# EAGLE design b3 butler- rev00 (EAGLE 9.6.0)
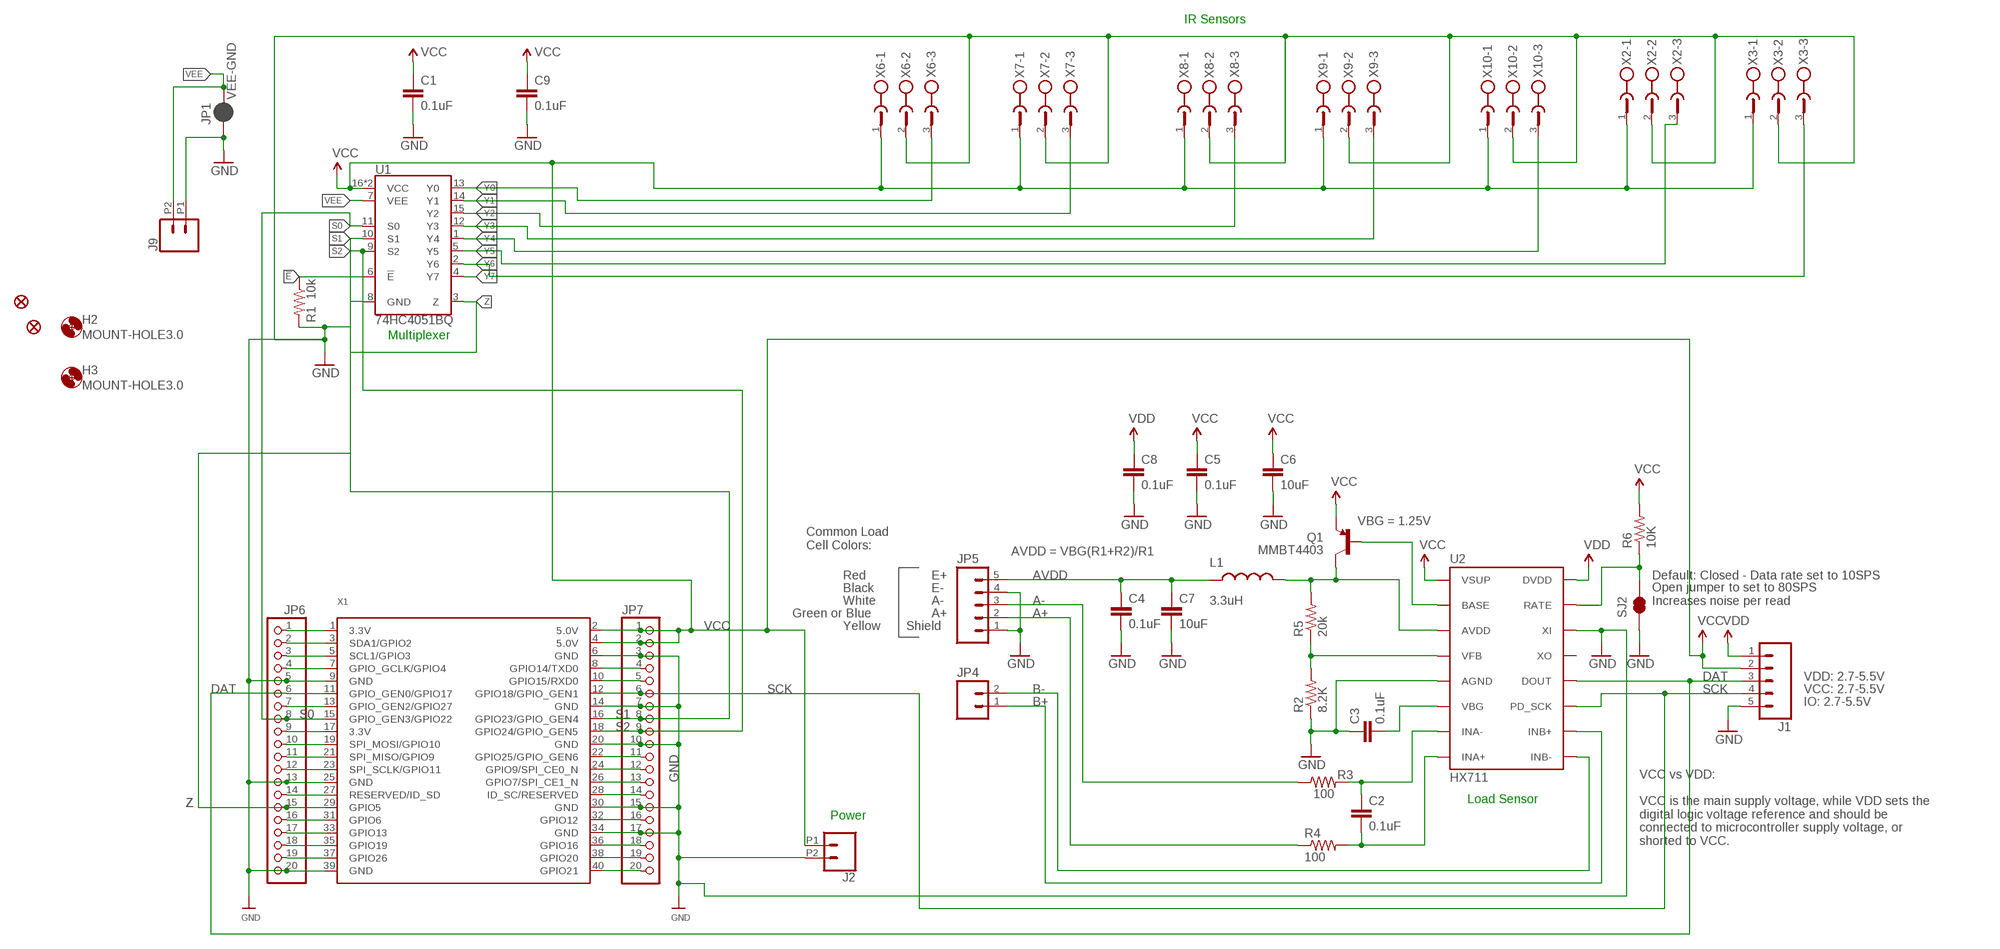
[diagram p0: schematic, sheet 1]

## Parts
C1  0.1uF  0.1UF-0603-25V-(+80/-20%)  [0603]
C2  0.1uF  0.1UF-25V-5%(0603)  [0603-CAP]
C3  0.1uF  0.1UF-25V-5%(0603)  [0603-CAP]
C4  0.1uF  0.1UF-25V-5%(0603)  [0603-CAP]
C5  0.1uF  0.1UF-25V-5%(0603)  [0603-CAP]
C6  10uF  10UF50V20%(1210)  [1210]
C7  10uF  10UF50V20%(1210)  [1210]
C8  0.1uF  0.1UF-25V-5%(0603)  [0603-CAP]
C9  0.1uF  0.1UF-0603-25V-(+80/-20%)  [0603]
FD1  FIDUCIAL1X2  [FIDUCIAL-1X2]
FD2  FIDUCIAL1X2  [FIDUCIAL-1X2]
H2  MOUNT-HOLE3.0  [3,0]
H3  MOUNT-HOLE3.0  [3,0]
J1  M05PTH  [1X05]
J2  CONN_022.54MM_SCREWTERM  [1X02_2.54_SCREWTERM]
J9  CONN_022.54MM_SCREWTERM  [1X02_2.54_SCREWTERM]
JP1  VEE-GND  JUMPER-PAD-2-NC_BY_PASTENO-SILK  [PAD-JUMPER-2-NC_BY_PASTE_NO_SILK]
JP4  M02PTH  [1X02@1]
JP5  M05PTH  [1X05]
JP6  HEADER-1X20ROUND  [1X20_ROUND]
JP7  HEADER-1X20ROUND  [1X20_ROUND]
L1  3.3uH  INDUCTOR0805-IND  [0805]
Q1  MMBT4403  TRANSISTOR_PNPMMBT4403  [SOT23-3]
R1  10k  10KOHM-0603-1/10W-1%  [0603]
R2  8.2K  8.2KOHM-1/10W-5%(0603)  [0603-RES]
R3  100  100OHM-1/10W-1%(0603)  [0603-RES]
R4  100  100OHM-1/10W-1%(0603)  [0603-RES]
R5  20k  20KOHM1/10W1%(0603)  [0603-RES]
R6  10K  10KOHM-1/10W-1%(0603)0603  [0603-RES]
SJ2  JUMPER-PAD-2-NC_BY_TRACE  [PAD-JUMPER-2-NC_BY_TRACE_YES_SILK]
U1  74HC4051BQ  [DHVQFN-16-2.5X3.5MM]
U2  HX711  HX711HX711  [SO16]
X1  RASPBERRYPI_B+_IDC  [RASPBERRYPI_B+_IDC]
X2  W232-3  [W232-3]
X3  W232-3  [W232-3]
X6  W232-3  [W232-3]
X7  W232-3  [W232-3]
X8  W232-3  [W232-3]
X9  W232-3  [W232-3]
X10  W232-3  [W232-3]

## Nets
!E!: R1.1 U1.6(!E!)
A+: JP5.2 R4.1
A-: JP5.3 R3.1
AVDD [POWER]: C4.1 C7.1 JP5.5 L1.1
B+: JP4.1 U2.10(INB+)
B-: JP4.2 U2.9(INB-)
DAT: J1.3 JP6.6 U2.12(DOUT) X1.11(GPIO_GEN0/GPIO17)
GND [POWER]: C1.2 C3.1 C4.2 C5.2 C6.2 C7.2 C8.2 C9.2 J1.5 J2.P2 J9.P1 JP1.1 JP5.1 JP5.4 JP6.5 JP6.13 JP6.20 JP7.3 JP7.7 JP7.10 JP7.15 JP7.17 R1.2 R2.1 SJ2.1 U1.8(GND) U2.5(AGND) U2.14(XI) X1.6(GND) X1.9(GND) X1.14(GND) X1.20(GND) X1.25(GND) X1.30(GND) X1.34(GND) X1.39(GND) X2.2 X3.2 X6.2 X7.2 X8.2 X9.2 X10.2
N$1: R6.1 SJ2.2 U2.15(RATE)
N$2: C2.1 R3.2 U2.7(INA-)
N$3: C2.2 R4.2 U2.8(INA+)
N$4: Q1.1(B) U2.2(BASE)
N$5: L1.2 Q1.3(C) R5.2 U2.3(AVDD)
N$6: R2.2 R5.1 U2.4(VFB)
N$7: C3.2 U2.6(VBG)
N$11: JP7.4 X1.8(GPIO14/TXD0)
N$12: JP7.5 X1.10(GPIO15/RXD0)
N$16: JP7.11 X1.22(GPIO25/GPIO_GEN6)
N$17: JP7.12 X1.24(GPIO9/SPI_CE0_N)
N$18: JP7.13 X1.26(GPIO7/SPI_CE1_N)
N$19: JP7.14 X1.28(ID_SC/RESERVED)
N$20: JP7.16 X1.32(GPIO12)
N$21: JP7.18 X1.36(GPIO16)
N$22: JP7.19 X1.38(GPIO20)
N$23: JP7.20 X1.40(GPIO21)
N$24: JP6.1 X1.1(3.3V)
N$25: JP6.2 X1.3(SDA1/GPIO2)
N$26: JP6.3 X1.5(SCL1/GPIO3)
N$27: JP6.4 X1.7(GPIO_GCLK/GPIO4)
N$29: JP6.7 X1.13(GPIO_GEN2/GPIO27)
N$31: JP6.9 X1.17(3.3V)
N$32: JP6.10 X1.19(SPI_MOSI/GPIO10)
N$33: JP6.11 X1.21(SPI_MISO/GPIO9)
N$34: JP6.12 X1.23(SPI_SCLK/GPIO11)
N$35: JP6.14 X1.27(RESERVED/ID_SD)
N$37: JP6.16 X1.31(GPIO6)
N$38: JP6.17 X1.33(GPIO13)
N$39: JP6.18 X1.35(GPIO19)
N$40: JP6.19 X1.37(GPIO26)
S0: JP6.8 U1.11(S0) X1.15(GPIO_GEN3/GPIO22)
S1: JP7.8 U1.10(S1) X1.16(GPIO23/GPIO_GEN4)
S2: JP7.9 U1.9(S2) X1.18(GPIO24/GPIO_GEN5)
SCK: J1.4 JP7.6 U2.11(PD_SCK) X1.12(GPIO18/GPIO_GEN1)
VCC [IR SENSORS]: C1.1 C5.1 C6.1 C9.1 J1.2 J2.P1 JP7.1 JP7.2 Q1.2(E) R6.2 U1.16(VCC) U1.EP(VCC) U2.1(VSUP) X1.2(5.0V) X1.4(5.0V) X2.1 X3.1 X6.1 X7.1 X8.1 X9.1 X10.1
VDD [POWER]: C8.1 J1.1 U2.16(DVDD)
VEE [POWER]: J9.P2 JP1.2 U1.7(VEE)
Y0 [IR SENSORS]: U1.13(Y0) X6.3
Y1 [IR SENSORS]: U1.14(Y1) X7.3
Y2 [IR SENSORS]: U1.15(Y2) X8.3
Y3 [IR SENSORS]: U1.12(Y3) X9.3
Y4 [IR SENSORS]: U1.1(Y4) X10.3
Y5 [IR SENSORS]: U1.5(Y5) X2.3
Y6 [IR SENSORS]: U1.2(Y6) X3.3
Y7 [IR SENSORS]: U1.4(Y7)
Z: JP6.15 U1.3(Z) X1.29(GPIO5)
Unconnected: U2.13(XO)

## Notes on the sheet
- IR Sensors
- Multiplexer
- VBG = 1.25V
- Common Load
  Cell Colors:
- AVDD = VBG(R1+R2)/R1
- Red | E+ | Default: Closed - Data rate set to 10SPS
- Black | E-
- White | A-
- Open jumper to set to 80SPS
  Increases noise per read
- Green or Blue | A+
- Yellow | Shield
- VDD: 2.7-5.5V
- VCC: 2.7-5.5V
- IO: 2.7-5.5V
- Load Sensor
- Power
- VCC vs VDD:
  
  VCC is the main supply voltage, while VDD sets the
  digital logic voltage reference and should be
  connected to microcontroller supply voltage, or
  shorted to VCC.

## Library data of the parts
C1 C9 = SparkFun-Capacitors:0.1UF: 0.1µF ceramic capacitors; PROD_ID: CAP-00810
C2-C5 C8 = SparkFun-Capacitors:0.1UF-25V-5%(0603): CAP-08604; PROD_ID: CAP-08604
C6 C7 = SparkFun-Capacitors:10UF50V20%(1210): CAP-09824; PROD_ID: CAP-09824
FD1 FD2 = SparkFun-Aesthetics:FIDUCIAL: Fiducial Alignment Points
H2 H3 = holes:MOUNT-HOLE: MOUNTING HOLE with drill center marker
J1 JP5 = SparkFun-Connectors:M05: Header 5 Standard 5-pin 0.1" header. Use with straight break away headers (SKU : PRT-00116), right angle break away headers (PRT-00553), swiss pins (PRT-00743), machine pins (PRT-00117), and female headers (PRT-00115). Molex polarized connector foot print use with SKU : PRT-08230 with associated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
J2 J9 = SparkFun-Connectors:CONN_02: Multi connection point. Often used as Generic Header-pin footprint for 0.1 inch spaced/style header connections
JP1 = SparkFun-Passives:JUMPER-PAD-2-NC_BY_PASTE
JP4 = SparkFun-Connectors:M02: Standard 2-pin 0.1" header. Use with
JP6 JP7 = microbuilder:HEADER-1X20
L1 = SparkFun-Passives:INDUCTOR: Inductors; PROD_ID: NDUC-13076
Q1 = SparkFun-DiscreteSemi:TRANSISTOR_PNP: Generic PNP BJT Double check pinouts against datasheets- not all devices are the same! MMBT3906 - 40V 200mA SOT-23 (TRANS-08052) MMBT4403 - 40V 600mA SOT-23 (TRANS-09245); PROD_ID: TRANS-09245
R1 = SparkFun-Resistors:10KOHM: 10kΩ resistor; PROD_ID: RES-00824
R2 = SparkFun-Resistors:8.2KOHM-1/10W-5%(0603): RES-10646; PROD_ID: RES-10646
R3 R4 = SparkFun-Resistors:100OHM-1/10W-1%(0603): RES-07863; PROD_ID: RES-07863
R5 = SparkFun-Resistors:20KOHM1/10W1%(0603): RES-09383; PROD_ID: RES-09383
R6 = SparkFun-Resistors:10KOHM-1/10W-1%(0603): RES-00824; PROD_ID: RES-00824
SJ2 = SparkFun-Passives:JUMPER-PAD-2-NC_BY_TRACE
U1 = 8mux:74HC4051: NXP 74HC4051 8-Channel Analog Multiplexer/Demultiplexer The 74HC4051; 74HCT4051 is a single-pole octal-throw analog switch (SP8T) suitable for use in analog or digital 8:1 multiplexer/demultiplexer applications. The switch features three digital select inputs (S0, S1 and S2), eight independent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; PROD_ID: IC-13334
U2 = Testing:HX711; PROD_ID: IC-12445
X1 = microbuilder:RASPBERRYPI_B+_IDC
X2 X3 X6-X10 = con-wago-508:W232-3: WAGO SREW CLAMP; OC_FARNELL: unknown; OC_NEWARK: unknown

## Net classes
0 default: width 0.203 mm, drill 0.406 mm, clearance 0.203 mm
1 POWER: width 0.813 mm, drill 0.406 mm, clearance 0.203 mm
2 IR SENSORS: width 0.203 mm, drill 0.203 mm, clearance 0.152 mm

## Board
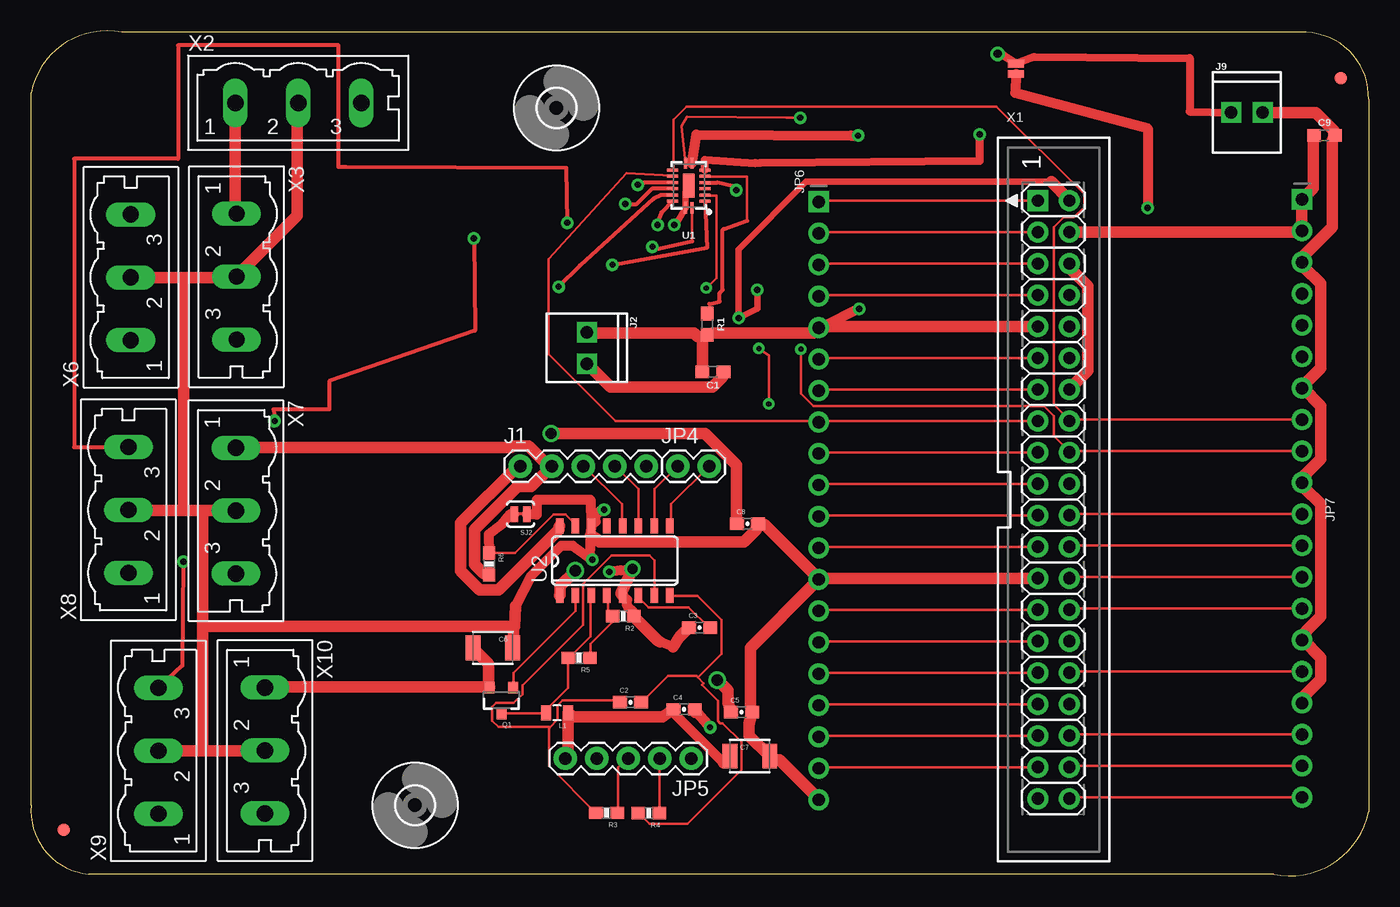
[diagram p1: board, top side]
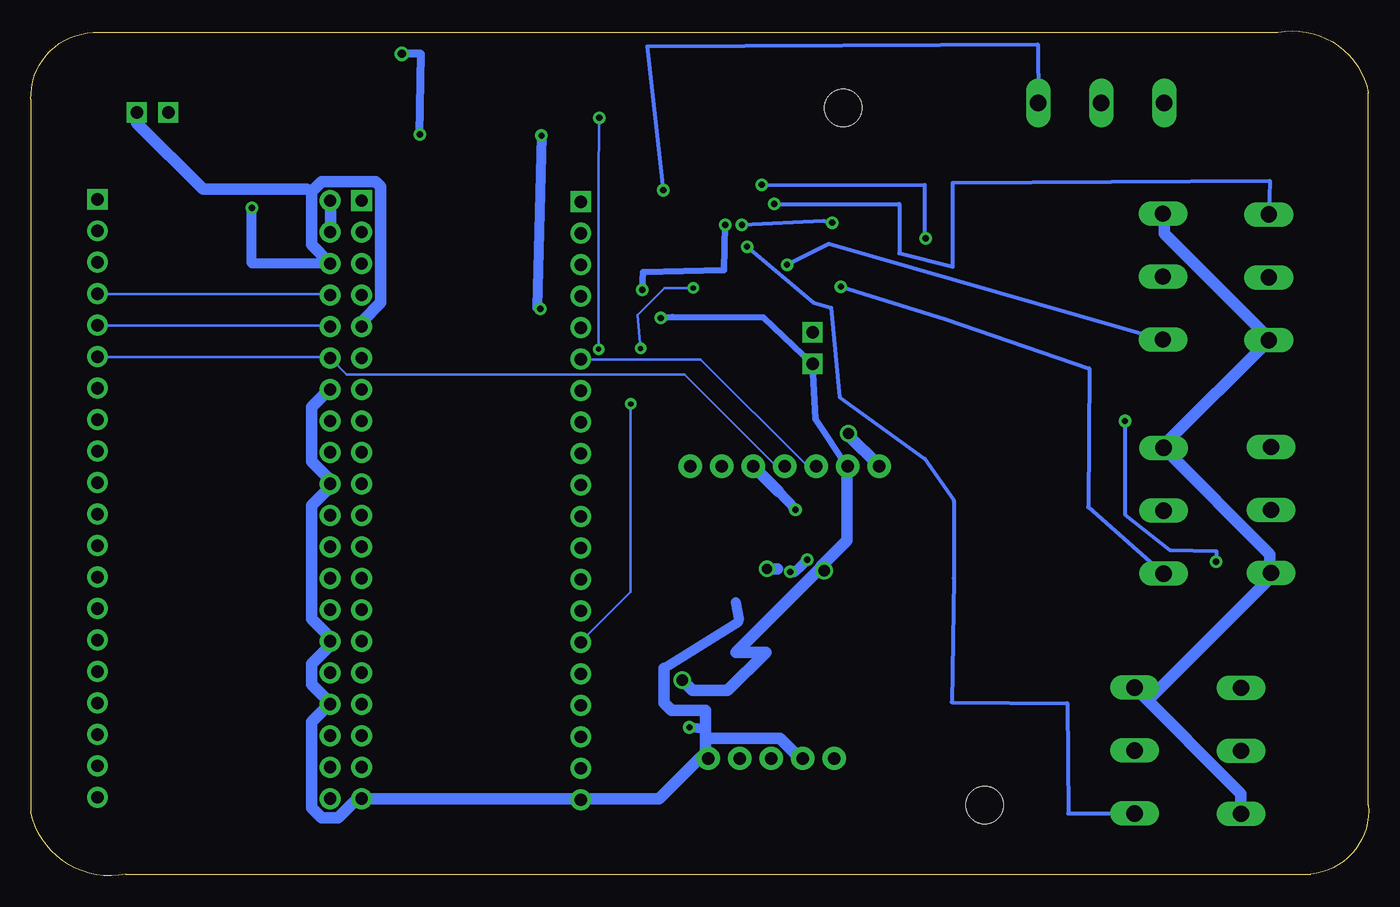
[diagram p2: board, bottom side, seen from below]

Size 107.91 x 68.17 mm. Coordinates in mm from the lower left corner, seen from the top.
Outline: 107.91,62.65 107.91,5.15 arc-90 100.26,0.13 4.66,0.13 arc-90 0.02,5.7 0.02,63.2 arc-90 7.3,68.05 102.9,68.05 arc-90 107.91,62.65
Copper layers (1*16): Top 0.035mm / dielectric 1.5mm / Bottom 0.035mm
Design rules "SparkFun": minimum track width 8mil, minimum drill 20mil, track to track 8mil, track to pad 8mil, pad to pad 8mil, via to via 8mil, smd to smd 8mil, copper to edge 8mil, drill to drill 8mil, minimum pad ring 12mil, minimum via ring 10mil, stop-mask expansion 4mil, vias tented up to drill 20mil, thermal gap 10mil

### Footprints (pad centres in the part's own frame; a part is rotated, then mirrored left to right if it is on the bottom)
0603 = smd 1.1 x 1: 1 -0.85,0; 2 0.85,0
0603-CAP = smd 1.1 x 1: 1 -0.85,0; 2 0.85,0
1210 = smd 1.2 x 2: 1 -1.6,0; 2 1.6,0
FIDUCIAL-1X2 = smd 1 x 1: 1 0,0
3,0 = hole 3: 0,0
1X05 = drill 1.016 pad 1.88: 1 0,0; 2 2.54,0; 3 5.08,0; 4 7.62,0; 5 10.16,0
1X02_2.54_SCREWTERM = drill 1.016 square: P1 2.54,0; P2 0,0
PAD-JUMPER-2-NC_BY_PASTE_NO_SILK = smd 0.635 x 1.27: 1 -0.401,0; 2 0.413,0
1X02@1 = drill 1.016 pad 1.88: 1 0,0; 2 2.54,0
1X20_ROUND = drill 1 pad 1.676 square: 1 -24.13,0 | drill 1 pad 1.676: 2 -21.59,0; 3 -19.05,0; 4 -16.51,0; 5 -13.97,0; 6 -11.43,0; 7 -8.89,0; 8 -6.35,0; 9 -3.81,0; 10 -1.27,0; 11 1.27,0; 12 3.81,0; 13 6.35,0; 14 8.89,0; 15 11.43,0; 16 13.97,0; 17 16.51,0; 18 19.05,0; 19 21.59,0; 20 24.13,0
0805 = smd 0.8 x 1.2: 1 -0.9,0; 2 0.9,0
SOT23-3 = smd 0.8 x 0.9: 1 -0.95,-1; 2 0.95,-1; 3 0,1.1
0603-RES = smd 1.1 x 1: 1 -0.85,0; 2 0.85,0
PAD-JUMPER-2-NC_BY_TRACE_YES_SILK = smd 0.635 x 1.27: 1 -0.508,0; 2 0.508,0
DHVQFN-16-2.5X3.5MM = smd 0.9 x 0.24: 1 -1.8,-0.25; 8 1.8,-0.25; 9 1.8,0.25; 16 -1.8,0.25 | smd 0.24 x 0.9: 2 -1.25,-1.3; 3 -0.75,-1.3; 4 -0.25,-1.3; 5 0.25,-1.3; 6 0.75,-1.3; 7 1.25,-1.3; 10 1.25,1.3; 11 0.75,1.3; 12 0.25,1.3; 13 -0.25,1.3; 14 -0.75,1.3; 15 -1.25,1.3 | smd 1.9 x 0.9: EP 0,0
SO16 = smd 0.6 x 1.2: 1 -4.445,-2.8; 2 -3.175,-2.8; 3 -1.905,-2.8; 4 -0.635,-2.8; 5 0.635,-2.8; 6 1.905,-2.8; 7 3.175,-2.8; 8 4.445,-2.8; 9 4.445,2.8; 10 3.175,2.8; 11 1.905,2.8; 12 0.635,2.8; 13 -0.635,2.8; 14 -1.905,2.8; 15 -3.175,2.8; 16 -4.445,2.8
RASPBERRYPI_B+_IDC = drill 1 pad 1.676 square: 1 -1.27,24.13 | drill 1 pad 1.676: 2 1.27,24.13; 3 -1.27,21.59; 4 1.27,21.59; 5 -1.27,19.05; 6 1.27,19.05; 7 -1.27,16.51; 8 1.27,16.51; 9 -1.27,13.97; 10 1.27,13.97; 11 -1.27,11.43; 12 1.27,11.43; 13 -1.27,8.89; 14 1.27,8.89; 15 -1.27,6.35; 16 1.27,6.35; 17 -1.27,3.81; 18 1.27,3.81; 19 -1.27,1.27; 20 1.27,1.27; 21 -1.27,-1.27; 22 1.27,-1.27; 23 -1.27,-3.81; 24 1.27,-3.81; 25 -1.27,-6.35; 26 1.27,-6.35; 27 -1.27,-8.89; 28 1.27,-8.89; 29 -1.27,-11.43; 30 1.27,-11.43; 31 -1.27,-13.97; 32 1.27,-13.97; 33 -1.27,-16.51; 34 1.27,-16.51; 35 -1.27,-19.05; 36 1.27,-19.05; 37 -1.27,-21.59; 38 1.27,-21.59; 39 -1.27,-24.13; 40 1.27,-24.13
W232-3 = drill 1.321 long: 1 -5.08,-0.635; 2 0,-0.635; 3 5.08,-0.635

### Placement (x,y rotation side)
C1  55.02,40.67 180 top
C2  48.37,14 0 top
C3  53.94,20.03 0 top
C4  52.69,13.43 0 top
C5  57.33,13.2 0 top
C6  37.26,18.38 0 top
C7  58,9.66 0 top
C8  57.81,28.41 0 top
C9  104.35,59.73 0 top
FD1  105.65,64.37 0 top
FD2  2.65,3.72 0 top
H2  42.4,61.96 0 top
H3  30.98,5.69 0 top
J1  39.48,33.05 0 top
J2  44.85,43.85 270 top
J9  96.83,61.59 0 top
JP1  79.46,65.11 90 top
JP4  52.18,33.05 0 top
JP5  53.26,9.47 180 top
JP6  63.55,30.26 270 top
JP7  102.55,30.46 270 top
L1  42.44,13.15 180 top
Q1  37.95,14.19 180 top
R1  54.57,44.51 270 top
R2  47.79,20.94 180 top
R3  46.44,5.08 180 top
R4  49.85,5.06 180 top
R5  44.22,17.59 180 top
R6  36.96,25.17 270 top
SJ2  39.5,29.18 180 top
U1  53.07,55.69 90 top
U2  47.1,25.43 0 top
X1  82.5,30.35 0 top
X2  21.57,63 0 top
X3  17.22,48.35 270 top
X6  7.41,48.29 90 top
X7  17.17,29.46 270 top
X8  7.22,29.52 90 top
X9  9.64,10.08 90 top
X10  19.52,10.11 270 top

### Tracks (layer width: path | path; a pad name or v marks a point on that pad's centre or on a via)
!E!
  Top 0.203: 57.77,52.85 57.77,56.41 54.39,56.41 U1.6 | R1.1 54.73,45.53 54.73,46.15
  Top 0.305: 54.73,46.15 55.55,46.35 55.55,47.01 55.8,47.27 55.8,52.11 55.89,52.19 57.77,52.85
A+
  Top 0.203: R4.1 50.73,5.1 JP5.2
A-
  Top 0.203: R3.1 47.37,5.1 47.37,8.76 48.09,9.47 JP5.3
AVDD
  Top 0.813: C4.1 51.84,13.15 55.86,9.12
  Top 0.914: C7.1 55.86,9.12 | JP5.5 43.11,9.57 43.31,9.77 43.31,13.13 L1.1 43.72,12.82 50.93,12.82 C4.1
B+
  Top 0.203: U2.10 50.32,28.26 50.32,31.21 52.15,33.04 JP4.1
B-
  Top 0.203: U2.9 51.64,28.26 51.64,29.99 54.69,33.04 JP4.2
DAT
  Top 0.203: U2.12 47.68,28.26 47.68,29.99 44.63,33.04 J1.3 | JP6.6 63.63,41.78 81.21,41.78 X1.11
  Bottom 0.203: J1.3 44.63,33.14 45.34,33.14 53.88,41.67 63.53,41.67 JP6.6
GND  (via drill 0.51, 0.81)
  Top 0.813: v90.09,53.89 90.09,60.32 79.42,63.18 JP1.1 | SJ2.1 40.82,29.15 40.82,30.35 45.13,30.35 U2.14 | 51.78,18.49 50.6,18.95 | R2.1 48.64,21.23 48.09,21.78 48.09,22.27 U2.5 | U2.14 45.16,27.65 | 45.16,27.65 45.05,25.78 v45.28,25.5 43.7,26.63 42.78,26.63 40.36,24.21 39.08,21.79 | v46.65,24.52 46.73,24.52 47.58,24.65 v48.53,24.77 | U2.14 45.55,28.59 45.55,29.08 45.91,29.44 46.13,29.44 v46.24,29.54 | 45.14,27.45 45.16,27.65 | C4.2 v54.79,11.98 | U1.8 53.69,59.81 66.13,59.73 v66.72,59.73 | v66.81,45.76 63.94,44.32
  Top 0.914: J9.P1 99.39,61.59 103.66,61.59 105.19,60.06 105.19,59.76 C9.2 104.98,59.35 104.98,52.34 102.65,50.01 102.65,49.6 JP7.3 102.75,49.09 104.07,47.77 104.07,40.96 102.85,39.74 JP7.7 102.65,39.34 104.07,37.92 104.07,33.65 102.65,32.23 102.65,31.82 JP7.10 102.75,31.31 104.07,29.99 104.07,20.95 102.85,19.73 102.85,19.42 JP7.15 102.65,19.02 104.07,17.6 104.07,15.87 102.65,14.45 102.65,14.04 JP7.17 | 54.18,43.3 54.18,40.76 C1.2 | 54.18,43.3 54.49,43.61 R1.2 54.99,43.81 63.12,43.81 63.53,44.21 JP6.5 63.94,44.32 81.21,44.32 X1.9 | J2.P2 44.94,43.81 53.47,43.81 53.78,43.5 54.18,43.3 | X1.6 83.85,49.4 83.85,48.99 85.27,47.57 85.27,40.76 83.85,39.34 X1.14 | 12.32,48.28 16.49,48.28 X3.2 16.89,48.69 21.47,53.26 21.47,62.3 X2.2 | 12.32,48.28 X6.2 | 13.85,10.08 18.83,10.08 X10.2 | 13.85,10.08 10.29,10.08 X9.2 | 13.85,29.48 16.49,29.48 X7.2 | 13.85,29.48 12.32,29.48 | 12.32,29.48 7.95,29.48 X8.2 | 13.85,29.48 13.85,20.14 | 13.85,20.14 13.85,10.08 | 12.32,29.48 12.32,48.28 | 50.73,18.88 50.6,18.95 48.7,20.85 R2.1 | C3.1 52.33,19.27 51.78,18.49 | v48.53,24.77 47.6,22.77 U2.5 | JP6.20 63.53,6.22 60.38,9.37 59.97,9.37 C7.2 59.57,9.67 57.94,11.3 57.94,12.27 C5.2 58.04,13.67 58.04,18.41 63.22,23.59 JP6.13 | 53.58,13.2 53.54,13.25 C4.2 | 38.94,20.14 38.94,18.41 C6.2 | 39.08,21.79 39.02,20.14 38.94,20.14 | JP6.13 63.53,24 59.16,28.37 58.75,28.37 C8.2 58.55,27.96 57.53,26.94 45.85,26.94 45.55,27.25 45.14,27.45 | X1.25 81.21,24 63.94,24 JP6.13 | 38.94,20.14 13.85,20.14
  Bottom 0.813: X1.6 90.09,49.4 v90.09,53.89 | 51.05,22.08 50.81,20.61 50.97,20.4 56.82,16.73 | v45.28,25.5 46.32,24.51 v46.65,24.52 | v46.24,29.54 47.6,31.02 | v54.79,11.98 53.47,11.9 | v66.72,59.73 67.06,45.84 v66.81,45.76
  Bottom 0.914: X1.14 83.85,39.24 85.27,37.81 85.27,33.45 83.85,32.02 83.85,31.72 X1.20 83.95,31.21 85.27,29.89 85.27,20.75 84.05,19.53 84.05,19.32 X1.30 83.85,18.92 83.85,18.51 85.27,17.09 85.27,15.46 84.05,14.24 X1.34 83.85,13.84 85.27,12.41 85.27,5.51 84.46,4.69 83.14,4.69 81.61,6.22 81.31,6.22 X1.39 80.8,6.22 63.94,6.22 JP6.20 63.53,6.22 57.23,6.22 53.88,9.57 JP5.1 53.27,9.57 53.47,9.77 53.47,11.09 | 85.27,55.19 84.46,56 80.09,56 79.68,55.59 79.68,46.25 81.21,44.72 81.21,44.42 X1.9 | 85.27,55.19 85.27,50.92 83.85,49.5 X1.6 | J9.P1 99.37,60.73 94.03,55.39 85.68,55.39 85.27,55.19 | 47.6,31.02 49.61,33.04 J1.5 | 48.38,24.75 47.68,24.75 v48.53,24.77 | 53.47,11.09 53.47,11.9 53.47,13.33 56.21,13.33 56.82,13.94 56.82,16.73 | 53.47,11.09 47.48,11.09 45.95,9.57 45.65,9.57 JP5.4
N$1
  Top 0.203: R6.1 37.04,26.03 39.05,26.03 42.17,29.15 43.14,29.15 44.02,28.26 U2.15
  Top 0.813: SJ2.2 38.67,29.18 37.91,28.29 36.92,27.56 R6.1
N$2
  Top 0.203: 41.84,11.96 42.5,12.62 42.5,13.73 42.9,14.14 47.37,14.14 47.48,14.04 C2.1 | 41.84,11.96 41.79,11.91 41.79,8.86 45.55,5.1 R3.2 | U2.7 50.32,22.68 50.32,25.44 49.9,25.86 46.83,25.86 44.53,23.56 44.53,20.24 39.65,15.36 39.65,14.65 38.94,13.94 37.52,13.94 37.21,13.63 37.21,12.52 37.72,12.01 41.79,12.01 41.84,11.96
N$3
  Top 0.203: 53.8,16.01 53.69,16.11 51.38,16.11 49.31,14.04 C2.2 | 53.8,16.01 54.26,15.54 54.13,15.41 55.42,14.13 55.42,12.5 55.6,12.31 55.81,12.31 57.33,10.79 57.33,8.55 52.96,4.18 49.91,4.18 49.1,5 R4.2 | 53.8,16.01 55.71,17.92 55.71,20.64 53.78,22.57 51.64,22.57 U2.8
N$4
  Top 0.203: Q1.1 38.94,15.26 38.94,16.38 43.92,21.35 43.92,22.57 U2.2
N$5
  Top 0.203: Q1.3 38.03,13.13 41.48,13.13 L1.2 41.58,13.23 41.58,13.43 43.31,15.16 43.31,17.49 R5.2 43.41,17.6 45.14,19.32 45.14,22.57 U2.3
N$6
  Top 0.203: R5.1 45.14,17.6 45.14,18.71 46.87,20.44 46.87,20.85 R2.2 46.87,20.95 46.56,21.25 46.56,22.57 U2.4
N$7
  Top 0.203: C3.2 54.69,20.03 53.06,21.66 49.81,21.66 49.1,22.37 49.1,22.57 U2.6
N$11
  Bottom 0.203: X1.8 83.85,46.96 JP7.4
N$12
  Bottom 0.203: X1.10 83.85,44.42 JP7.5
N$16
  Top 0.203: X1.22 83.85,29.18 JP7.11
N$17
  Top 0.203: X1.24 83.85,26.64 JP7.12
N$18
  Top 0.203: X1.26 83.85,24.1 JP7.13
N$19
  Top 0.203: X1.28 83.85,21.56 JP7.14
N$20
  Top 0.203: X1.32 83.85,16.48 JP7.16
N$21
  Top 0.203: X1.36 83.85,11.4 JP7.18
N$22
  Top 0.203: X1.38 83.85,8.86 JP7.19
N$23
  Top 0.203: X1.40 83.85,6.32 JP7.20
N$24
  Top 0.203: JP6.1 63.63,54.48 81.21,54.48 X1.1
N$25
  Top 0.203: JP6.2 63.63,51.94 81.21,51.94 X1.3
N$26
  Top 0.203: JP6.3 63.63,49.4 81.21,49.4 X1.5
N$27
  Top 0.203: JP6.4 63.63,46.86 81.21,46.86 X1.7
N$29
  Top 0.203: JP6.7 63.63,39.24 81.21,39.24 X1.13
N$31
  Top 0.203: JP6.9 63.63,34.16 81.21,34.16 X1.17
N$32
  Top 0.203: JP6.10 63.63,31.62 81.21,31.62 X1.19
N$33
  Top 0.203: JP6.11 63.63,29.08 81.21,29.08 X1.21
N$34
  Top 0.203: JP6.12 63.63,26.54 81.21,26.54 X1.23
N$35
  Top 0.203: JP6.14 63.63,21.46 81.21,21.46 X1.27
N$37
  Top 0.203: JP6.16 63.63,16.38 81.21,16.38 X1.31
N$38
  Top 0.203: JP6.17 63.63,13.84 81.21,13.84 X1.33
N$39
  Top 0.203: JP6.18 63.63,11.3 81.21,11.3 X1.35
N$40
  Top 0.203: JP6.19 63.63,8.76 81.21,8.76 X1.37
S0
  Top 0.203: U1.11 51.72,56.49 48.03,56.71 41.75,49.78 41.75,42.09 47.15,36.7 63.53,36.7 JP6.8 63.63,36.7 81.21,36.7 X1.15
S1
  Top 0.203: U1.10 51.85,57.02 51.85,58.71 51.85,61 52.9,62.06 77.89,62.06 84.97,54.98 84.97,53.97 84.15,53.16 83.34,53.16 82.53,52.34 82.53,38.02 83.75,36.8 X1.16 83.85,36.8 JP7.8
S2  (via drill 0.41, 0.51)
  Top 0.203: v62.11,42.49 62.11,38.93 63.12,37.92 81.72,37.92 82.53,37.1 82.53,35.48 83.75,34.26 X1.18 83.85,34.26 JP7.9 | U1.9 52.5,60.49 52.92,61.25 60.97,61.17 v62.07,61.17
  Bottom 0.203: 62.11,55.83 62.11,55.75 | 62.11,55.75 v62.11,42.49 | v62.07,61.17 62.11,55.75
SCK
  Top 0.203: U2.11 49,28.26 49,31.21 47.17,33.04 J1.4
  Bottom 0.203: JP7.6 83.85,41.88 X1.12 83.75,41.78 82.43,40.46 55.2,40.46 47.88,33.14 47.17,33.14 J1.4
VCC  (via drill 0.51, 0.91)
  Top 0.508: 82.33,56 62.51,56 57.06,50.55 v57.09,45.01 58.6,45.76 v58.6,47.28 | U1.EP 52.87,55.49 52.82,55.11 U1.16 52.16,52.79 v51.91,52.53
  Top 0.914: 36.91,15.26 36.91,17.09 35.69,18.31 C6.1 | 36.91,15.26 Q1.2 | 36.91,15.26 18.93,15.26 X10.1 | X3.1 16.49,53.46 16.49,62.3 X2.1 | C9.1 103.46,59.66 103.46,55.49 102.65,54.68 JP7.1 102.54,54.17 102.54,52.14 JP7.2 102.14,51.94 83.85,51.94 X1.4 | C1.1 55.81,40.66 55.81,40.25 54.99,39.44 46.77,39.44 44.94,41.27 J2.P1 | v55.37,15.8 56.21,14.95 56.21,14.01 C5.1 | R6.2 36.91,24.4 36.5,24.4 35.79,25.11 35.79,27.96 39.25,31.41 40.36,31.41 41.99,33.04 J1.2 41.58,33.24 40.16,34.66 38.84,34.66 38.74,34.56 16.59,34.56 X7.1 | v43.92,24.61 42.7,23.39 42.7,22.68 U2.1 | 82.33,56 83.75,54.58 X1.2
  Bottom 0.508: v57.09,45.01 56.16,45.07 48.8,45.05 44.83,41.27 | v51.91,52.53 51.99,48.89 58.51,48.72 v58.6,47.28 | J2.P1 44.63,36.87 42.09,33.04
  Bottom 0.914: X9.1 10.29,5.1 10.29,6.62 18.83,15.16 X10.1 17.5,14.45 7.95,24 X8.1 7.95,24.5 7.95,25.93 16.49,34.46 X7.1 16.39,34.87 X6.1 8.26,43.61 16.49,51.83 16.49,53.36 X3.1 | X1.4 83.75,52.04 83.75,54.48 X1.2 | v55.37,15.8 54.52,14.95 51.7,14.95 48.63,18.02 51.03,18.02 44.18,24.87 | v43.92,24.61 44.18,24.87 | 44.18,24.87 44.23,24.91 42.09,27.04 42.09,33.04 J1.2 42.29,33.45 | 44.83,41.27 J2.P1
VDD  (via drill 0.86)
  Top 0.914: v41.96,35.68 54.39,35.68 56.93,33.14 56.93,28.47 C8.1 | U2.16 42.6,28.16 42.6,27.96 37.72,23.08 36.2,23.08 34.67,24.61 34.67,28.47 39.25,33.04 39.45,33.04 J1.1
  Bottom 0.914: v41.96,35.68 41.96,35.55 39.55,33.14 J1.1
VEE  (via drill 0.51, 0.66)
  Top 0.66: v76.54,59.81 76.54,57.7 58.85,57.53 58.42,57.52 54.36,57.78 U1.7 | 78.2,66.33 JP1.2 80.95,66.08 93.47,65.99 93.47,61.67 J9.P2
  Top 0.813: 78.2,66.33 v77.98,66.33
  Bottom 0.66: v76.54,59.81 76.44,66.33 v77.98,66.33
Y0  (via drill 0.51)
  Top 0.305: U1.13 50.09,55.44 48.87,54.22 v47.93,54.22
  Bottom 0.305: v47.93,54.22 37.85,54.22 37.85,50.25 33.54,49.14 33.54,55.92 7.97,56.09 X6.3
Y1  (via drill 0.51)
  Top 0.305: U1.14 50.82,54.94 50.24,54.62 44.28,49.25 v42.57,47.54
  Bottom 0.305: v42.57,47.54 34.13,44.91 22.53,40.93 22.62,29.76 X7.3
Y2  (via drill 0.51)
  Top 0.305: U1.15 50.85,53.52 50.55,52.75 v50.55,52.53 | v43.27,52.7 43.28,52.71 43.19,57.11 25.41,57.19 24.82,57.19 24.82,67.01 11.86,67.01 11.86,57.86 3.48,57.86 3.48,34.58 X8.3
  Bottom 0.305: v50.55,52.53 43.96,52.86 v43.27,52.7
Y3  (via drill 0.51)
  Top 0.305: U1.12 49.45,55.92 v48.94,55.76 | v35.74,51.43 35.82,43.98 24.06,39.92 24.06,37.63 19.57,37.63 v19.65,36.7 | v12.29,25.36 12.2,16.97 X9.3
  Bottom 0.305: v48.94,55.76 35.82,55.75 35.82,51.77 v35.74,51.43 | v19.65,36.7 19.65,29.17 16.01,26.29 12.29,26.2 v12.29,25.36
Y4  (via drill 0.51)
  Top 0.203: U1.1 53.35,51.18
  Top 0.305: 53.35,51.18 50.64,50.58 v50.14,50.76
  Bottom 0.305: v50.14,50.76 44.8,46.27 43.36,45.84 42.68,38.65 35.82,33.65 33.45,30.27 33.45,24 33.62,14.01 24.31,13.93 24.22,5.04 X10.3
Y5  (via drill 0.51)
  Top 0.305: v56.9,55.32 56.6,55.63 55.38,55.94 U1.5
  Bottom 0.305: v56.9,55.32 56.88,55.35 58.17,66.92 26.68,67.09 X2.3
Y6  (via drill 0.51)
  Top 0.305: U1.2 54.53,50.67 47.25,49.31 v46.91,49.31
  Bottom 0.305: v46.91,49.31 43.53,51.01 X3.3
Z  (via drill 0.41)
  Top 0.203: v54.48,47.43 55.29,48.25 55.29,54.88 54.39,54.88 U1.3 | v59.52,38.07 59.52,41.98 v58.73,42.56 | X1.29 81.21,18.92 63.63,18.92 JP6.15
  Bottom 0.203: v58.73,42.56 58.97,45.26 56.81,47.43 v54.48,47.43 | v59.52,38.07 59.52,22.93 63.53,18.92 JP6.15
